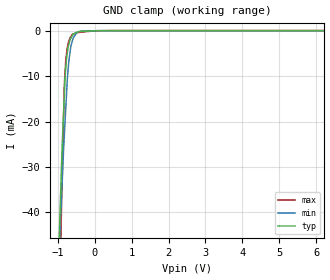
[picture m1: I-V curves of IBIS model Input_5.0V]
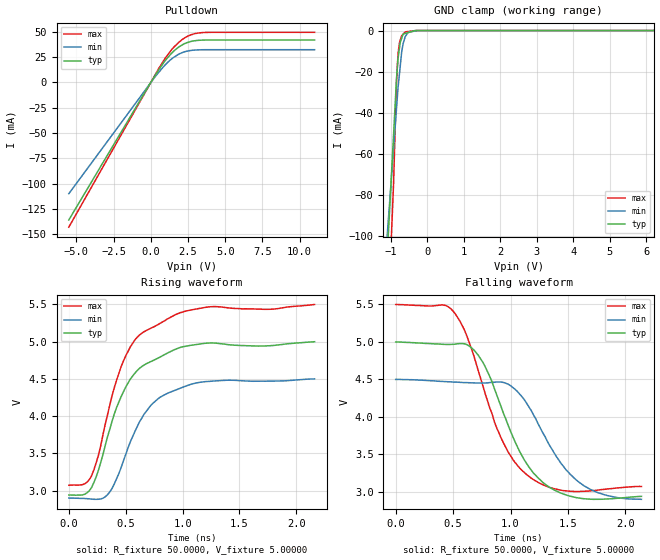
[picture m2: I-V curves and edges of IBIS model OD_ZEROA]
[IBIS Ver]   3.2
[Comment Char] |_char
[File Name]   pcm1755dbq.ibs
[File Rev]   3.0
[Source]
| This model file was created by Teraspeed Consulting Group LLC
| (http://www.teraspeed.com/).
[Date]   08-12-2004
[Notes]   Quality Check of this IBIS model: Model Passes IBIS Check
   Model parses into ICX IS. Simulation done with Hyperlynx.
   1. MIN TYP MAX information is based on Temprature and Voltage
   characteristics only.
[Disclaimer]
| This model is designed as an aid for customers of Texas Instruments.
| TI and its licensors and suppliers make no warranties, either expressed
| or implied, with respect to this  model, including the warranties of
| merchantability or fitness for a particular purpose.
| The model is provided solely on an "as is" basis. The entire risk as to
| its quality and performance is with the customer.
[Copyright]
| (C) Copyright 2008 Texas Instruments Incorporated. All rights reserved.
[Component] PCM1755DBQ
[Manufacturer] TI
[Package]
| variable   typ   min   max
R_pkg  1.8006E-02  1.8006E-02  1.8006E-02
L_pkg  2.1607E-09  2.1607E-09  2.1607E-09
C_pkg  6.0021E-13  6.0021E-13  6.0021E-13
[Pin] signal_name  model_name  R_pin  L_pin C_pin
1   BCK   Input_5.0V  1.7205E-02  2.4087E-09  4.9156E-13
2   DATA   Input_5.0V  1.6401E-02  2.2962E-09  4.6861E-13
3   LRCK   Input_5.0V  1.5620E-02  2.1869E-09  4.4630E-13
4   DGND   GND   1.4866E-02  2.0812E-09  4.2474E-13
5   NC   NC   1.4866E-02  2.0812E-09  4.2474E-13
6   VCC   POWER   1.5620E-02  2.1869E-09  4.4630E-13
7   VoutL   NC   1.6401E-02  2.2962E-09  4.6861E-13
8   VoutR   NC   1.7205E-02  2.4087E-09  4.9156E-13
9   AGND   GND   1.7205E-02  2.4087E-09  4.9156E-13
10  Vcom   POWER   1.6401E-02  2.2962E-09  4.6861E-13
11  ZEROR/ZEROA  OD_ZEROA   1.5620E-02  2.1869E-09  4.4630E-13
12  ZEROL/NA   OD_ZEROA   1.4866E-02  2.0812E-09  4.2474E-13
13  MD   Input_5.0V  1.4866E-02  2.0812E-09  4.2474E-13
14  MC   Input_5.0V  1.5620E-02  2.1869E-09  4.4630E-13
15  ML   Input_5.0V  1.6401E-02  2.2962E-09  4.6861E-13
16  SCK   Input_5.0V  1.7205E-02  2.4087E-09  4.9156E-13
| Models and submodels in the file (2): Input_5.0V (Input), OD_ZEROA (Open_sink)
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[Model] Input_5.0V
Model_type Input
Vinl  = 800.000mV
Vinh  = 2.00000V
C_comp  2.00000pF 2.00000pF 2.00000pF
| variable   typ   min   max
[Voltage Range]   5.00000V  4.50000V  5.50000V
[POWER Clamp Reference]  5.00000V  4.50000V  5.50000V
[GND Clamp Reference]   0.00000V  0.00000V  0.00000V
[Temperature Range]   25   85   -25
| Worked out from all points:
|   GND clamp passes 1 mA (typ) near -0.60 V on its own axis
[GND Clamp]
-5V       -1.087A    -810mA     -1.517A
-880.9mV  -25.98mA   -33.89mA   -33.7mA
-820.5mV  -14.28mA   -23.21mA   -11.95mA
-800.2mV  -10.35mA   -20.09mA   -9.142mA
-780.1mV  -8.211mA   -17.01mA   -6.379mA
-739.5mV  -4.822mA   -10.77mA   -3.65mA
-699.2mV  -2.997mA   -6.769mA   -2.216mA
-643.4mV  -1.576mA   -3.358mA   -1.226mA
-582.4mV  -754.1uA   -1.596mA   -686.4uA
-521.8mV  -381.3uA   -827.4uA   -492.1uA
-144.7mV  -4.114uA   57.5uA     -83.98uA
10V       78.15uA    57.5uA     92.87uA
[POWER Clamp]
| Voltage   I(typ)   I(min)   I(max)
-5.5V     0A         0A         0A
-5.4V     0A         0A         0A
-5.3V     0A         0A         0A
11V       0A         0A         0A
[Model] OD_ZEROA
Model_type Open_sink
Vref  = 5.00000V
Rref  = 50.0000ohms
Cref  = 2.00000pF
Vmeas = 4.50000V
C_comp  2.00000pF 2.00000pF 2.00000pF
[Model Spec]
Vmeas  4.4000V  4.3000V  4.5000V
| variable   typ   min   max
[Voltage Range]   5.00000V  4.50000V  5.50000V
[POWER Clamp Reference]  5.00000V  4.50000V  5.50000V
[Pulldown Reference]   0.00000V  0.00000V  0.00000V
[GND Clamp Reference]   0.00000V  0.00000V  0.00000V
[Temperature Range]   25   85   -25
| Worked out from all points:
|   slope of the pulldown table from 0 to 0.75 V, typ, clamps not added: 44.1 ohm
|   GND clamp passes 1 mA (typ) near -0.52 V on its own axis
|   falling waveform, R_fixture 50.0000, V_fixture 5.00000: 20-80 % time 347ps typ, 388ps min, 335ps max; typ from 5 V to 2.94 V
|   rising waveform, R_fixture 50.0000, V_fixture 5.00000: 20-80 % time 312ps typ, 307ps min, 303ps max; typ from 2.94 V to 5 V
[GND Clamp]
-5.5V     -1.603A    -1.169A    -2.065A
-4.5V     -1.264A    -926.2mA   -1.63A
-921.4mV  -50.58mA   -57.41mA   -74.31mA
-840.7mV  -23.22mA   -37.82mA   -24.88mA
-800.2mV  -13.76mA   -27.98mA   -11.49mA
-759.8mV  -8.457mA   -20.93mA   -5.878mA
-739.5mV  -5.795mA   -17.4mA    -4.74mA
-699.2mV  -3.772mA   -10.37mA   -2.48mA
-602.8mV  -1.441mA   -2.992mA   -656.5uA
-521.8mV  -1.014mA   -866.9uA   -480uA
-260.9mV  0A         0A         0A
11V       0A         0A         0A
[Pulldown]
-5.5V     -135.8mA   -109.9mA   -142.9mA
20.9mV    529uA      260.4uA    420.9uA
643.4mV   14.82mA    11.88mA    16.31mA
982.2mV   21.74mA    17.57mA    24.19mA
1.381V    28.6mA     23.02mA    31.96mA
1.882V    35.05mA    27.96mA    39.65mA
2.14V     37.35mA    29.64mA    42.75mA
2.822V    40.92mA    31.86mA    47.7mA
3.58V     41.9mA     32.37mA    49.42mA
11V       41.96mA    32.39mA    49.55mA
[POWER Clamp]
| Voltage   I(typ)   I(min)   I(max)
-5.5V     0A         0A         0A
-5.4V     0A         0A         0A
-5.3V     0A         0A         0A
11V       0A         0A         0A
[Falling Waveform]
R_fixture = 50.0000
V_fixture = 5.00000
V_fixture_min = 4.50000
V_fixture_max = 5.50000
0s        5V         4.5V       5.5V
420ps     4.968V     4.472V     5.492V
520ps     4.972V     4.464V     5.372V
620ps     4.965V     4.457V     5.08V
760ps     4.727V     4.452V     4.411V
980ps     3.885V     4.436V     3.529V
1.18ns    3.291V     4.085V     3.183V
1.4ns     3.01V      3.469V     3.035V
1.58ns    2.921V     3.149V     3.005V
2.14ns    2.94V      2.9V       3.072V
[Rising Waveform]
R_fixture = 50.0000
V_fixture = 5.00000
V_fixture_min = 4.50000
V_fixture_max = 5.50000
0s        2.94V      2.9V       3.072V
120ps     2.942V     2.895V     3.079V
200ps     3.041V     2.886V     3.198V
260ps     3.272V     2.884V     3.474V
340ps     3.723V     2.944V     4.017V
480ps     4.327V     3.4V       4.74V
640ps     4.665V     3.97V      5.113V
800ps     4.792V     4.252V     5.245V
1.12ns    4.962V     4.446V     5.439V
2.16ns    5V         4.5V       5.5V
[Ramp]
| variable  typ   min   max
dV/dt_r   706.701m/326.348p  556.472m/326.268p  830.654m/307.716p
dV/dt_f   1.23679/347.202p   959.917m/388.409p  1.45689/335.384p
R_load = 50.0000Ohms
